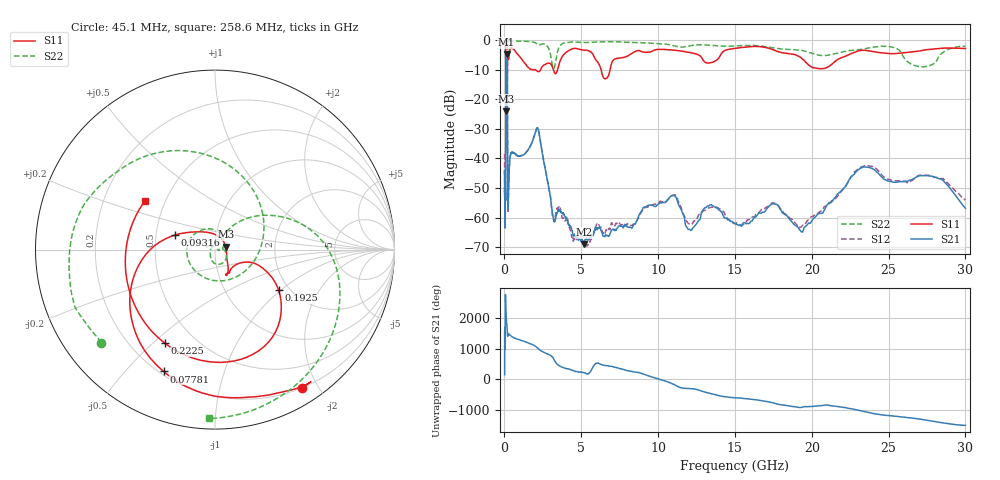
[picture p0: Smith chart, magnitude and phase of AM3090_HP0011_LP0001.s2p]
! Date/Time: Thu, Feb 28, 2019 1:56 PM
! Network Analyzer: Agilent Technologies E8364B Rev: A.07.50.67
! Sweep from 0.010 to 30.000 GHz, 1601 Points, Sweep Type: LOG
! Power Supply: 5.023 V, 0.002 A
# Hz S DB R 50
!freq MagS11 AngS11 MagS21 AngS21 MagS12 AngS12 MagS22 AngS22
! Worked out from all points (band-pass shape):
!   1601 points, 10 MHz to 30 GHz, reference 50 ohm
!   highest |S21| = -4.76 dB at 137.6 MHz (marker M1); lowest = -69.0 dB at 5.18 GHz (marker M2)
!   |S21| within 3 dB of the highest: 101.2 MHz to 177.8 MHz (76.62 MHz wide, 54.9 % of centre)
!   lowest |S11| = -24.1 dB at 100.4 MHz (marker M3), VSWR 1.13, Z = 56.4 + j1.83 ohm
!   |S11| at or under -10 dB: 1.995 GHz to 2.353 GHz (357.6 MHz wide, 16.5 % of centre); 3.186 GHz to 3.459 GHz (273.3 MHz wide, 8.23 % of centre); 6.288 GHz to 6.876 GHz (588.1 MHz wide, 8.93 % of centre)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
!   |S22| runs from -36.9 to -0.1 dB; largest |S21 - S12| = 0.017
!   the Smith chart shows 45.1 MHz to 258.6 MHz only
!   S11 on the Smith chart (normalised r, x): 45.1 MHz: 0.20, -1.79; 77.81 MHz: 0.22, -0.64; 93.16 MHz: 0.63, +0.11; 192.5 MHz: 1.76, -0.97; 222.5 MHz: 0.34, -0.55; 258.6 MHz: 0.39, +0.27
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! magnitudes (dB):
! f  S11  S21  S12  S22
! 10 MHz  -0.2  -45.1  -38.4  -0.5
! 38.04 MHz  -0.5  -62.0  -60.6  -1.3
! 45.1 MHz  -0.8  -54.1  -53.3  -1.7
! 77.81 MHz  -2.7  -46.4  -46.3  -5.2
! 93.16 MHz  -12.5  -14.1  -14.2  -15.5
! 100.4 MHz  -24.1  -8.1  -8.1  -16.6
! 127.7 MHz  -16.4  -4.9  -4.9  -36.6
! 137.6 MHz  -16.5  -4.8  -4.7  -28.0
! 144.7 MHz  -16.3  -4.8  -4.8  -22.6
! 170.7 MHz  -15.8  -6.4  -6.4  -33.4
! 192.5 MHz  -7.5  -17.6  -17.7  -10.4
! 222.5 MHz  -4.6  -55.1  -57.5  -1.4
! 258.6 MHz  -6.5  -52.6  -53.7  -0.5
! 550.5 MHz  -3.0  -38.0  -38.1  -0.2
! 2.084 GHz  -10.3  -30.0  -30.0  -1.2
! 3.204 GHz  -10.3  -60.8  -60.4  -9.6
! 5.18 GHz  -3.4  -69.0  -68.8  -0.8
! 7.926 GHz  -5.6  -62.4  -62.2  -0.7
! 10.81 GHz  -3.3  -52.8  -52.9  -1.7
! 19.41 GHz  -6.4  -64.8  -62.5  -3.6
! 23.48 GHz  -3.5  -42.9  -42.3  -2.9
! 30 GHz  -2.9  -56.9  -54.0  -2.1
